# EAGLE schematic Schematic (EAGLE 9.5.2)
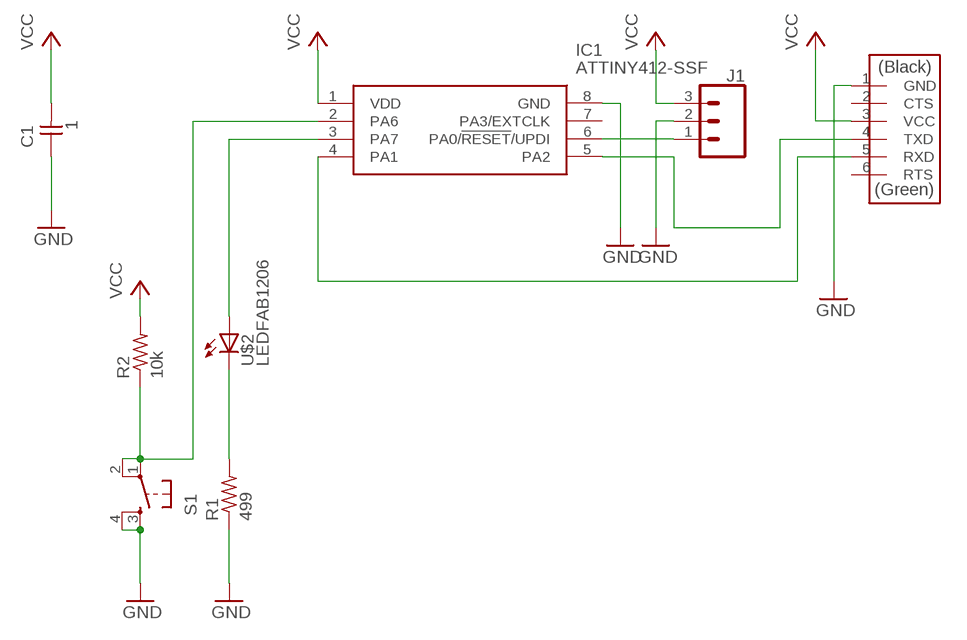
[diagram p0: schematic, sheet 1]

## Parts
C1  1  CAP_UNPOLARIZEDFAB  [C1206FAB]
IC1  ATTINY412-SSF  [SOIC127P600X175-8N]
J1  CONN_03SMD_RA_MALE  [1X03_SMD_RA_MALE]
R1  499  R1206FAB  [R1206FAB]
R2  10k  R1206FAB  [R1206FAB]
S1  SW_SWITCH_TACTILE_6MM6MM_SWITCH  [6MM_SWITCH]
U$1  CONN_06_FTDI-SMD-HEADER  [1X06SMD]
U$2  LEDFAB1206  [LED1206FAB]

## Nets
GND: C1.1 IC1.8(GND) J1.2 R1.1 S1.3(S) S1.4(S1) U$1.1(GND)
N$1: IC1.3(PA7) U$2.1(A)
N$2: IC1.4(PA1) U$1.5(RXD)
N$3: IC1.5(PA2) U$1.4(TXD)
N$4: IC1.2(PA6) R2.1 S1.1(P) S1.2(P1)
N$6: R1.2 U$2.2(C)
N$7: IC1.6(PA0/!RESET!/UPDI) J1.1
VCC: C1.2 IC1.1(VDD) J1.3 R2.2 U$1.3(VCC)
Unconnected: IC1.7(PA3/EXTCLK) U$1.2(CTS) U$1.6(RTS)

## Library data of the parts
C1 = fab:CAP_UNPOLARIZED
IC1 = ATTINY412-SSF:ATTINY412-SSF: 8-bit Microcontrollers - MCU 20MHz, 4KB, SOIC8, Ind 125C, Green, Tube Source: Datasheet; DESCRIPTION: 8-bit Microcontrollers - MCU 20MHz, 4KB, SOIC8, Ind 125C, Green, Tube; HEIGHT: 1.75mm; MANUFACTURER_NAME: Microchip; MANUFACTURER_PART_NUMBER: ATTINY412-SSF; MOUSER_PART_NUMBER: 579-ATTINY412-SSF; MOUSER_PRICE-STOCK: https://www.mouser.com/Search/Refine.aspx?Keyword=579-ATTINY412-SSF
J1 = SparkFun-Connectors:CONN_03: Multi connection point. Often used as Generic Header-pin footprint for 0.1 inch spaced/style header connections On any of the 0.1 inch spaced packages, you can populate with these: Break Away Headers - Straight (PRT-00116) Break Away Male Headers - Right Angle (PRT-00553) Female Headers (PRT-00115)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; PROD_ID: CONN-10925
R1 R2 = fab:R: Resistor (US Symbol)
S1 = fab:SW_SWITCH_TACTILE_6MM: OMRON SWITCH
U$1 = fab:CONN_06_FTDI-SMD-HEADER
U$2 = fab:LED: LED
